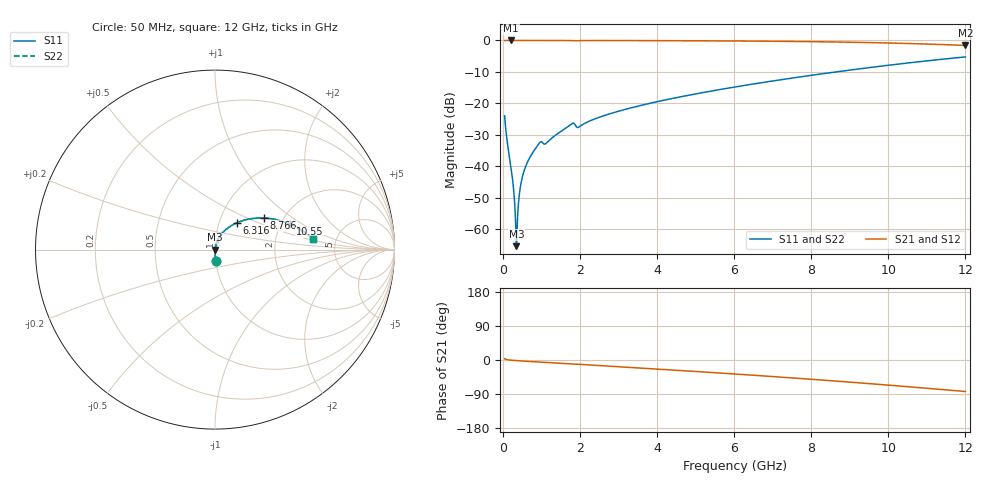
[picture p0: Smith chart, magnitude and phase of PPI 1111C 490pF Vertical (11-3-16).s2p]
# GHz S MA R 50
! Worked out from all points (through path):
!   1601 points, 50 MHz to 12 GHz, reference 50 ohm
!   highest |S21| = 0.00 dB at 221.8 MHz (marker M1); lowest = -1.6 dB at 12 GHz (marker M2)
!   group delay of S21, straight-line fit = 19.1 ps
!   lowest |S11| = -65.4 dB at 356.2 MHz (marker M3), VSWR 1.00, Z = 50.1 - j0.00518 ohm
!   |S11| at or under -10 dB: start of sweep to 8.645 GHz
!   |S22| runs from -65.4 to -5.2 dB; largest |S21 - S12| = 0
!   S11 on the Smith chart (normalised r, x): 50 MHz: 1.00, -0.13; 6.316 GHz: 1.22, +0.38; 8.766 GHz: 1.59, +0.63; 10.55 GHz: 2.24, +0.79; 12 GHz: 3.31, +0.58
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0.05  0.0635 -86.3  0.9977 3.4  0.9977 3.4  0.0635 -86.3
0.2217813  0.009011 -87.7  0.9995 -0.5  0.9995 -0.5  0.009011 -87.7
0.2665938  0.005419 -85.8  0.9995 -0.9  0.9995 -0.9  0.005419 -85.8
0.318875  0.002127 -77.4  0.9995 -1.3  0.9995 -1.3  0.002127 -77.4
0.3562187  0.0005383 -5.5  0.9994 -1.6  0.9994 -1.6  0.0005383 -5.5
0.3935625  0.001878 70.8  0.9994 -1.9  0.9994 -1.9  0.001878 70.8
0.4607812  0.004783 80.4  0.9994 -2.3  0.9994 -2.3  0.004783 80.4
0.5429375  0.008007 82.4  0.9993 -2.9  0.9993 -2.9  0.008007 82.4
0.677375  0.01287 82.8  0.9991 -3.8  0.9991 -3.8  0.01287 82.8
0.8865  0.02063 80.5  0.9982 -5.2  0.9982 -5.2  0.02063 80.5
1.132969  0.02337 75.6  0.9964 -6.4  0.9964 -6.4  0.02337 75.6
1.790219  0.04734 72.9  0.9935 -10.7  0.9935 -10.7  0.04734 72.9
2.044156  0.04484 73.9  0.9955 -11.7  0.9955 -11.7  0.04484 73.9
2.761156  0.0678 72.4  0.9959 -16.2  0.9959 -16.2  0.0678 72.4
4.038312  0.1075 64.9  0.9922 -24.1  0.9922 -24.1  0.1075 64.9
6.025  0.1822 52.4  0.9807 -36.9  0.9807 -36.9  0.1822 52.4
6.316281  0.195 50.4  0.9782 -38.9  0.9782 -38.9  0.195 50.4
8.019156  0.2801 38.5  0.9568 -50.9  0.9568 -50.9  0.2801 38.5
8.766031  0.3235 32.9  0.9428 -56.5  0.9428 -56.5  0.3235 32.9
10.01331  0.4039 23.2  0.9108 -66.4  0.9108 -66.4  0.4039 23.2
10.55106  0.4413 18.8  0.8932 -70.8  0.8932 -70.8  0.4413 18.8
12  0.5473 6.4  0.8321 -83.2  0.8321 -83.2  0.5473 6.4
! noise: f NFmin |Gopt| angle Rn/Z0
0.05  0.000352  0.8589  0.2672  0.0005338
1.372  0.004539  0.7225  6.065  0.003235
2.701  0.006519  0.6402  11.69  0.003387
4.031  0.008354  0.5967  17.07  0.003729
5.36  0.01036  0.5788  22.25  0.004316
6.682  0.01242  0.5724  27.19  0.004989
8.012  0.01462  0.5742  31.97  0.005786
9.341  0.01701  0.5829  36.57  0.006753
10.67  0.01968  0.5975  41.02  0.00796
12  0.02273  0.6174  45.37  0.009508
